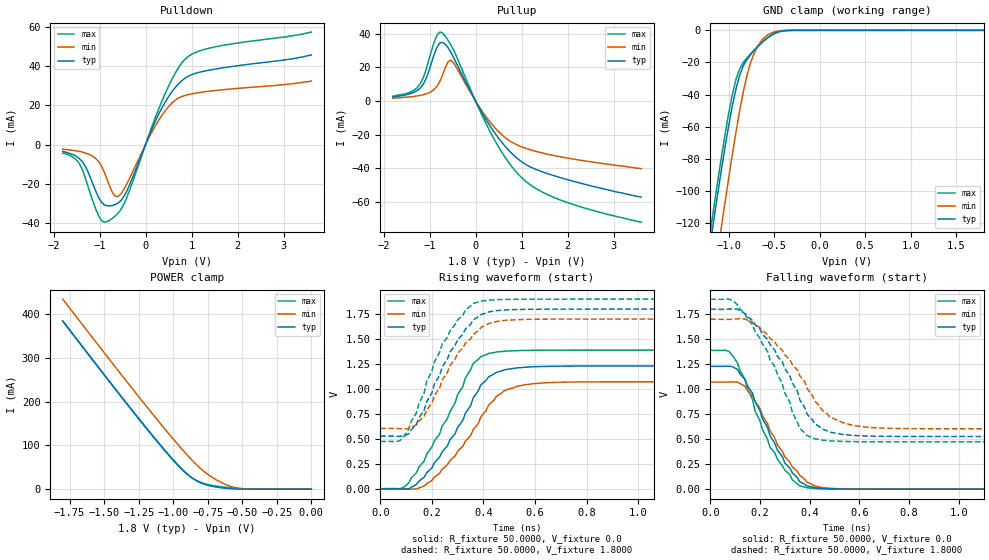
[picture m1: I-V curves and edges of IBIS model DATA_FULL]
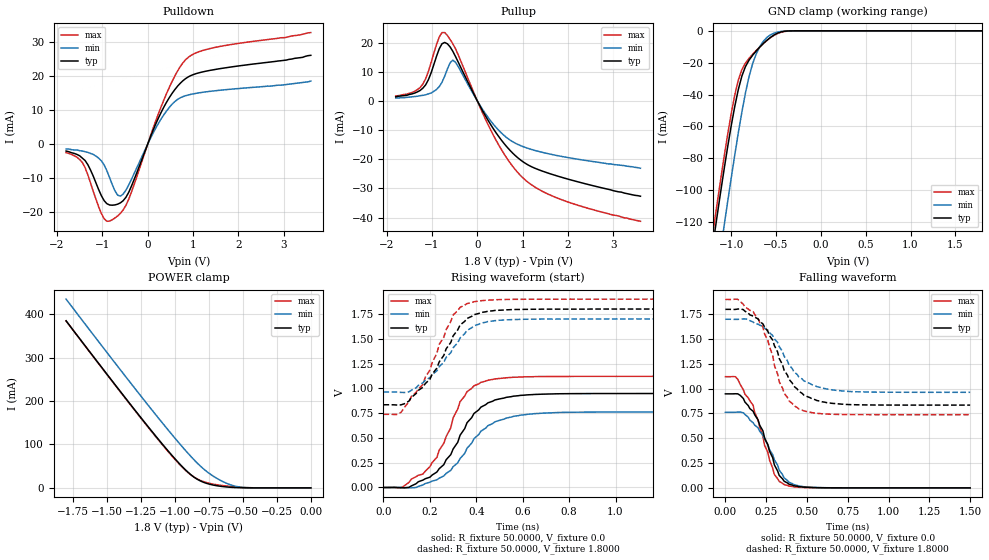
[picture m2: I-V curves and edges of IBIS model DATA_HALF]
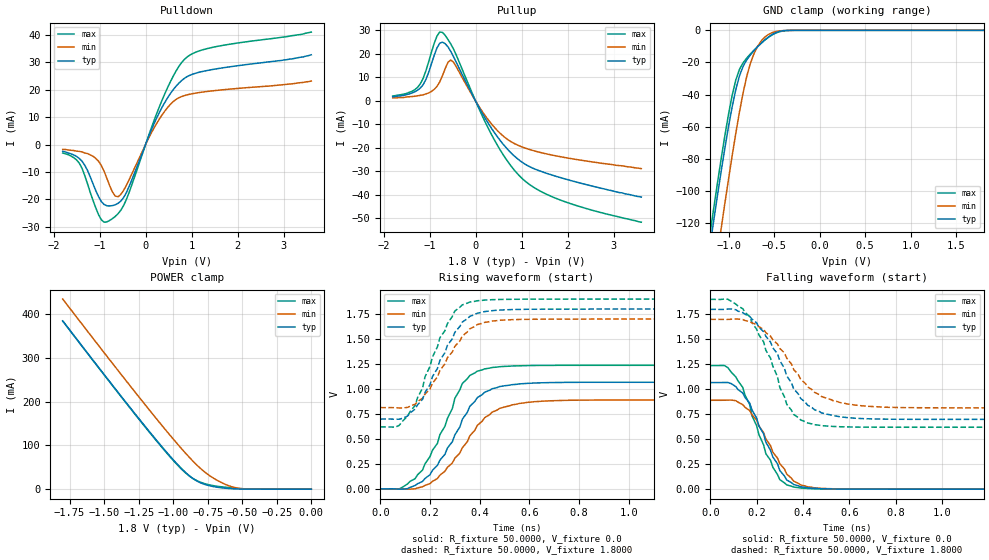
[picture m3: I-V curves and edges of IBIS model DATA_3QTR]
| IBIS file usesk1g16ac.ibs created by s2ibis3 verion 1.1
| North Carolina State University, ERL, 2006
| This Model is valid for Commercial Temperature Range 0C<=Tc<=70C
| Valid for LPDDR-333/400 operation
| Part Number   VDD/VDDQ   Package   Architecture
| SCE18K1G160AF   1.8 +0.1/-0.1  60-Ball FBGA   64Meg x 16
[IBIS Ver]   3.2
[File name]  usesk1g16ac.ibs
[File Rev]   1.2
[Date]   2015-10-27
[Source]   Simulation of a silicon level SPICE model
[Notes]   IBIS Characteristics for I/O Buffer
   IBIS Model Revision History:
Rev 1.1: 2015-10-27
   - IBIS model file initial creation
Rev 1.2: 2016-10-27
   - Updata company and other informations
[disclaimer] The IBIS models are for modeling purpose only and are
   subject to change without any notice. UniIC is not
   responsible for any problems the models may cause.
[Copyright]  Copyright 2015 UniIC Semiconductors Corp. All rights reserved
|   Component SCE18K1G160AF
[Component]   SCE18K1G160AF
[Manufacturer]  UniIC Semiconductors Corp.
| All balls excluding NC, POWER and GND (R[Ohm], L[H], C[F])
[Package]   | 60-Ball FBGA
|Variable   typ   min   max
R_pkg   366m   250m   672m
L_pkg   1.68n   1.12n   2.83n
C_pkg   0.31p   0.20p   0.55p
[Pin]   signal_name model_name   R_pin   L_pin   C_pin
A1   VSS   GND
A2   DQ15   DQ   374m   1.51n   0.32p
A3   VSSQ   GND
A7   VDDQ   POWER
A8   DQ0   DQ   390m   1.48n   0.35p
A9   VDD   POWER
B2   DQ13   DQ   444m   2n   0.4p
B3   DQ14   DQ   332m   1.35n   0.29p
B7   DQ1   DQ   268m   1.19n   0.25p
B8   DQ2   DQ   410m   1.6n   0.37p
B9   VSSQ   GND
C1   VSSQ   GND
C2   DQ11   DQ   370m   1.5n   0.34p
C3   DQ12   DQ   318m   1.58n   0.29p
C7   DQ3   DQ   294m   1.27n   0.28p
C8   DQ4   DQ   387m   1.66n   0.36p
C9   VDDQ   POWER
D1   VDDQ   POWER
D2   DQ9   DQ   391m   1.83n   0.33p
D3   DQ10   DQ   267m   1.14n   0.24p
D7   DQ5   DQ   250m   1.12n   0.27p
D8   DQ6   DQ   405m   1.87n   0.32p
D9   VSSQ   GND
E1   VSSQ   GND
E2   UDQS   DQ   406m   1.72n   0.37p
E3   DQ8   DQ   276m   1.28n   0.25p
E7   DQ7   DQ   275m   1.47n   0.21p
E8   LDQS   DQ   395m   1.59n   0.32p
E9   VDDQ   POWER
F1   VSS   GND
F2   UDM   DATA_RCV   388m   1.82n   0.32p
F7   A13   CLKCA_RCV   264m   1.18n   0.24p
F8   LDM   DATA_RCV   398m   1.54n   0.36p
F9   VDD   POWER
G1   CKE   CLKCA_RCV   453m   2.62n   0.36p
G2   CK   CLKCA_RCV   364m   1.97n   0.32p
G3   CK#   CLKCA_RCV   353m   1.72n   0.25p
G7   WE#   CLKCA_RCV   284m   1.32n   0.26p
G8   CAS#   CLKCA_RCV   381m   1.69n   0.35p
G9   RAS#   CLKCA_RCV   474m   2.32n   0.4p
H1   A9   CLKCA_RCV   457m   2.73n   0.33p
H2   A11   CLKCA_RCV   388m   2.17n   0.29p
H3   A12   CLKCA_RCV   263m   1.36n   0.25p
H7   CS#   CLKCA_RCV   262m   1.22n   0.24p
H8   BA0   CLKCA_RCV   394m   1.67n   0.36p
H9   BA1   CLKCA_RCV   508m   2.19n   0.42p
J1   A6   CLKCA_RCV   672m   2.79n   0.55p
J2   A7   CLKCA_RCV   380m   1.64n   0.3p
J3   A8   CLKCA_RCV   253m   1.34n   0.2p
J7   A10   CLKCA_RCV   263m   1.28n   0.22p
J8   A0   CLKCA_RCV   364m   1.68n   0.29p
J9   A1   CLKCA_RCV   661m   2.83n   0.54p
K1   VSS   GND
K2   A4   CLKCA_RCV   412m   1.87n   0.34p
K3   A5   CLKCA_RCV   266m   1.3n   0.23p
K7   A2   CLKCA_RCV   250m   1.18n   0.24p
K8   A3   CLKCA_RCV   367m   1.75n   0.31p
K9   VDD   POWER
|*****************************  Diff Pin  *************************************
[Diff Pin]  inv_pin  vdiff   tdelay_typ  tdelay_min  tdelay_max
G2   G3   1.08V   NA   NA   NA
|*****************************  Model Selector ********************************
[Model Selector]   DQ
DATA_FULL   Full-Strength Output Driver
DATA_3QTR   75% Strength Output Driver
DATA_HALF   Half-Strength Output Driver
DATA_RCV   Data/Data Strobe/Data Mask Receiver
| Models and submodels in the file (5): DATA_FULL (I/O), DATA_HALF (I/O), DATA_3QTR (I/O), DATA_RCV (Input), CLKCA_RCV (Input)
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|   Model DATA_FULL
[Model]  DATA_FULL
Model_type   I/O
Polarity   Non-Inverting
Enable   Active-High
Vinl  = 360.000mV
Vinh  = 1440.000mV
Vmeas = 900.000mV
Cref  = 20.000pF
C_comp   2.0990pF   2.0750pF   2.3110pF
[Temperature Range]   25.0000   70.0000   0.0
[Voltage Range]   1.8000V   1.7000V   1.9000V
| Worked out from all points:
|   slope of the pulldown table from 0 to 0.27 V, typ, clamps not added: 18.2 ohm
|   slope of the pullup table from 0 to 0.27 V, typ, clamps not added: 21 ohm
|   GND clamp passes 1 mA (typ) near -0.46 V on its own axis
|   POWER clamp passes 1 mA (typ) near -0.57 V on its own axis
|   rising waveform, R_fixture 50.0000, V_fixture 0.0: 20-80 % time 173ps typ, 179ps min, 160ps max; typ from 0 V to 1.23 V
|   rising waveform, R_fixture 50.0000, V_fixture 1.8000: 20-80 % time 150ps typ, 150ps min, 141ps max; typ from 0.527 V to 1.8 V
|   falling waveform, R_fixture 50.0000, V_fixture 0.0: 20-80 % time 143ps typ, 148ps min, 140ps max; typ from 1.23 V to 0 V
|   falling waveform, R_fixture 50.0000, V_fixture 1.8000: 20-80 % time 174ps typ, 187ps min, 158ps max; typ from 1.8 V to 0.527 V
[Pulldown]
|Voltage   I(typ)   I(min)   I(max)
-1.8V     -3.5mA     -2.4mA     -4.4mA
-1.44V    -7.2mA     -3.5mA     -9.6mA
-1.26V    -13.5mA    -4.7mA     -20.7mA
-1.02V    -27.06mA   -8.7mA     -36.42mA
-840mV    -31.35mA   -17.64mA   -39.44mA
-660mV    -30.74mA   -26.42mA   -36.6mA
-540mV    -28.79mA   -25.39mA   -33.36mA
360mV     18.94mA    15.09mA    22.48mA
660mV     29.6mA     22.96mA    37.15mA
900mV     34.59mA    25.38mA    44.54mA
1.56V     38.77mA    27.72mA    50.17mA
3.6V      45.8mA     32.5mA     57.5mA
[Pullup]
|Voltage   I(typ)   I(min)   I(max)
-1.8V     2.5mA      1.7mA      2.9mA
-1.26V    6.4mA      3.1mA      8.2mA
-1.08V    13.03mA    4.3mA      18.27mA
-840mV    31.99mA    8.72mA     39.09mA
-720mV    34.94mA    15.29mA    40.57mA
-600mV    31.88mA    23.25mA    36.23mA
-540mV    29.17mA    24.33mA    33.62mA
360mV     -16.7mA    -14.04mA   -20.48mA
720mV     -29.32mA   -23.3mA    -36.55mA
1.02V     -36.51mA   -27.44mA   -46.11mA
1.92V     -46.19mA   -33.57mA   -59.68mA
3.6V      -57.2mA    -40.3mA    -72.1mA
[GND_clamp]
|Voltage   I(typ)   I(min)   I(max)
-1.8V     -382.1mA   -420.9mA   -375.5mA
-1.2V     -133.2mA   -170.8mA   -125.6mA
-1.16V    -117.7mA   -154.8mA   -110mA
-1.08V    -87.61mA   -123.2mA   -79.77mA
-1V       -59.95mA   -92.78mA   -52.3mA
-920mV    -36.92mA   -64.12mA   -30.96mA
-880mV    -28.39mA   -50.93mA   -24.34mA
-800mV    -18.4mA    -28.71mA   -17.29mA
-680mV    -10.16mA   -9.871mA   -10.08mA
-560mV    -4.068mA   -2.483mA   -4.273mA
-320mV    -22.85uA   -25.25uA   -54.98uA
1.8V      3.312nA    24.23nA    3.394nA
[POWER_clamp]
|Voltage   I(typ)   I(min)   I(max)
-1.8V     384.7mA    434.6mA    384.4mA
-1.4V     221.6mA    271.6mA    220.8mA
-1.14V    119.1mA    168.3mA    117.7mA
-960mV    53.65mA    99.93mA    52.25mA
-900mV    35.09mA    78.55mA    34.34mA
-860mV    24.89mA    65.06mA    25.09mA
-800mV    14.21mA    46.71mA    15.61mA
-720mV    6.601mA    27.45mA    8.67mA
-640mV    2.692mA    13.43mA    5.023mA
-560mV    790.7uA    4.166mA    2.388mA
-440mV    59.56uA    254.6uA    284uA
0V        3.312nA    8.237nA    3.878nA
[Ramp]
| variable   typ   min   max
dV/dt_r  0.7374/0.1699n   0.6426/0.1795n   0.8334/0.1648n
dV/dt_f  0.7638/0.1717n   0.6576/0.1866n   0.8558/0.1598n
R_load = 50.0000
[Rising Waveform]
R_fixture= 50.0000
V_fixture= 0.0
V_fixture_min= 0.0
V_fixture_max= 0.0
|time   V(typ)   V(min)   V(max)
0s        0V         0V         0V
90.91ps   -4.216mV   -497.2uV   15.11mV
140ps     41.75mV    -2.255mV   158.6mV
170ps     115mV      26.85mV    275.9mV
290ps     551.3mV    327.8mV    860.2mV
360ps     908.9mV    590.6mV    1.254V
420ps     1.121V     838.2mV    1.355V
480ps     1.191V     980.7mV    1.378V
590ps     1.222V     1.052V     1.387V
1.5ns     1.229V     1.071V     1.389V
[Rising Waveform]
R_fixture= 50.0000
V_fixture= 1.8000
V_fixture_min= 1.7000
V_fixture_max= 1.9000
|time   V(typ)   V(min)   V(max)
0s        527mV      604mV      473.6mV
75.76ps   524.6mV    601.8mV    480.6mV
140ps     646.7mV    638.8mV    759.9mV
200ps     959.8mV    857mV      1.179V
240ps     1.22V      1.089V     1.452V
300ps     1.494V     1.357V     1.692V
360ps     1.69V      1.544V     1.855V
420ps     1.771V     1.655V     1.889V
520ps     1.794V     1.692V     1.897V
1.5ns     1.8V       1.7V       1.9V
[Falling Waveform]
R_fixture= 50.0000
V_fixture= 0.0
V_fixture_min= 0.0
V_fixture_max= 0.0
|time   V(typ)   V(min)   V(max)
0s        1.229V     1.071V     1.389V
75.76ps   1.231V     1.072V     1.377V
110ps     1.197V     1.07V      1.259V
170ps     959.1mV    934.7mV    898.6mV
180ps     877.9mV    875.6mV    781.7mV
240ps     535.2mV    582.8mV    419.7mV
300ps     261.6mV    322.9mV    189.5mV
360ps     74.58mV    138.3mV    32.52mV
480ps     4.177mV    8.446mV    1.931mV
1.5ns     0V         -795nV     0V
[Falling Waveform]
R_fixture= 50.0000
V_fixture= 1.8000
V_fixture_min= 1.7000
V_fixture_max= 1.9000
|time   V(typ)   V(min)   V(max)
0s        1.8V       1.7V       1.9V
90.91ps   1.805V     1.7V       1.884V
170ps     1.688V     1.669V     1.646V
290ps     1.273V     1.388V     1.053V
350ps     982.2mV    1.193V     673.8mV
360ps     894.7mV    1.136V     607mV
420ps     655.1mV    883.1mV    504.4mV
480ps     571.5mV    724.7mV    483.2mV
620ps     532.4mV    622mV      474.5mV
1.5ns     527mV      604mV      473.6mV
|   Model DATA_HALF
[Model]  DATA_HALF
Model_type   I/O
Polarity   Non-Inverting
Enable   Active-High
Vinl  = 360.000mV
Vinh  = 1440.000mV
Vmeas = 900.000mV
Cref  = 20.000pF
C_comp   2.0990pF   2.0750pF   2.3110pF
[Temperature Range]   25.0000   70.0000   0.0
[Voltage Range]   1.8000V   1.7000V   1.9000V
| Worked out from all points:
|   slope of the pulldown table from 0 to 0.27 V, typ, clamps not added: 31.3 ohm
|   slope of the pullup table from 0 to 0.27 V, typ, clamps not added: 36.1 ohm
|   GND clamp passes 1 mA (typ) near -0.46 V on its own axis
|   POWER clamp passes 1 mA (typ) near -0.57 V on its own axis
|   rising waveform, R_fixture 50.0000, V_fixture 0.0: 20-80 % time 156ps typ, 168ps min, 137ps max; typ from 0 V to 0.948 V
|   rising waveform, R_fixture 50.0000, V_fixture 1.8000: 20-80 % time 149ps typ, 150ps min, 145ps max; typ from 0.834 V to 1.8 V
|   falling waveform, R_fixture 50.0000, V_fixture 0.0: 20-80 % time 140ps typ, 145ps min, 140ps max; typ from 0.948 V to 0 V
|   falling waveform, R_fixture 50.0000, V_fixture 1.8000: 20-80 % time 172ps typ, 179ps min, 146ps max; typ from 1.8 V to 0.834 V
[Pulldown]
|Voltage   I(typ)   I(min)   I(max)
-1.8V     -2mA       -1.4mA     -2.5mA
-1.44V    -4.1mA     -2mA       -5.4mA
-1.02V    -15.18mA   -4.9mA     -20.41mA
-840mV    -17.9mA    -9.82mA    -22.65mA
-660mV    -17.64mA   -15.01mA   -21.1mA
-540mV    -16.62mA   -14.68mA   -19.34mA
-360mV    -12.42mA   -10.4mA    -14.2mA
300mV     9.454mA    7.512mA    11.15mA
600mV     16.1mA     12.58mA    20.1mA
840mV     19.36mA    14.31mA    24.93mA
1.44V     21.91mA    15.68mA    28.39mA
3.6V      26.2mA     18.6mA     32.9mA
[Pullup]
|Voltage   I(typ)   I(min)   I(max)
-1.8V     1.4mA      1mA        1.7mA
-1.38V    2.7mA      1.5mA      3.3mA
-1.2V     4.4mA      1.9mA      5.8mA
-1.08V    7.23mA     2.4mA      10.07mA
-840mV    17.87mA    4.9mA      21.91mA
-720mV    20.06mA    8.48mA     23.44mA
-600mV    18.52mA    13.08mA    21.06mA
-480mV    15.19mA    13.26mA    17.84mA
360mV     -9.695mA   -8.123mA   -11.94mA
1.02V     -21.01mA   -15.74mA   -26.6mA
1.86V     -26.2mA    -19.05mA   -33.89mA
3.6V      -32.7mA    -23.1mA    -41.3mA
[GND_clamp]
|Voltage   I(typ)   I(min)   I(max)
-1.8V     -382.1mA   -420.9mA   -375.5mA
-1.2V     -133.2mA   -170.8mA   -125.6mA
-1.16V    -117.7mA   -154.8mA   -110mA
-1.08V    -87.61mA   -123.2mA   -79.77mA
-1V       -59.95mA   -92.78mA   -52.3mA
-920mV    -36.92mA   -64.12mA   -30.96mA
-880mV    -28.39mA   -50.93mA   -24.34mA
-800mV    -18.4mA    -28.71mA   -17.29mA
-680mV    -10.16mA   -9.871mA   -10.08mA
-560mV    -4.068mA   -2.483mA   -4.273mA
-320mV    -22.85uA   -25.25uA   -54.98uA
1.8V      3.312nA    24.23nA    3.394nA
[POWER_clamp]
|Voltage   I(typ)   I(min)   I(max)
-1.8V     384.7mA    434.6mA    384.4mA
-1.4V     221.6mA    271.6mA    220.8mA
-1.14V    119.1mA    168.3mA    117.7mA
-960mV    53.65mA    99.93mA    52.25mA
-900mV    35.09mA    78.55mA    34.34mA
-860mV    24.89mA    65.06mA    25.09mA
-800mV    14.21mA    46.71mA    15.61mA
-720mV    6.601mA    27.45mA    8.67mA
-640mV    2.692mA    13.43mA    5.023mA
-560mV    790.7uA    4.166mA    2.388mA
-440mV    59.56uA    254.6uA    284uA
0V        3.312nA    8.237nA    3.878nA
[Ramp]
| variable   typ   min   max
dV/dt_r  0.5687/0.1549n   0.4570/0.1668n   0.6726/0.1381n
dV/dt_f  0.5793/0.1729n   0.4419/0.1794n   0.6973/0.1449n
R_load = 50.0000
[Rising Waveform]
R_fixture= 50.0000
V_fixture= 0.0
V_fixture_min= 0.0
V_fixture_max= 0.0
|time   V(typ)   V(min)   V(max)
0s        0V         0V         0V
75.76ps   -2.229mV   491.3uV    -1.644mV
200ps     103.9mV    53.19mV    210mV
260ps     230.8mV    117mV      446.2mV
330ps     527.3mV    292.8mV    866mV
360ps     653.7mV    396.5mV    967mV
420ps     811mV      568.5mV    1.061V
530ps     909.9mV    701mV      1.107V
650ps     938.4mV    744.7mV    1.118V
1.5ns     947.9mV    761.7mV    1.121V
[Rising Waveform]
R_fixture= 50.0000
V_fixture= 1.8000
V_fixture_min= 1.7000
V_fixture_max= 1.9000
|time   V(typ)   V(min)   V(max)
0s        834.5mV    963.5mV    737.9mV
75.76ps   833.5mV    959.1mV    758.7mV
170ps     1.011V     1.056V     1.039V
230ps     1.204V     1.176V     1.353V
240ps     1.267V     1.218V     1.444V
300ps     1.529V     1.41V      1.74V
360ps     1.705V     1.585V     1.855V
420ps     1.765V     1.658V     1.884V
530ps     1.792V     1.691V     1.897V
1.5ns     1.8V       1.7V       1.9V
[Falling Waveform]
R_fixture= 50.0000
V_fixture= 0.0
V_fixture_min= 0.0
V_fixture_max= 0.0
|time   V(typ)   V(min)   V(max)
0s        947.9mV    761.7mV    1.121V
60.61ps   948.9mV    762.2mV    1.121V
110ps     900.9mV    757mV      989.3mV
170ps     772.5mV    656.6mV    832.2mV
230ps     574.9mV    532.6mV    519.2mV
240ps     505.7mV    488.2mV    428.9mV
300ps     232mV      282.8mV    135.1mV
360ps     67.03mV    100.4mV    33.3mV
530ps     3.545mV    5.524mV    1.62mV
1.5ns     0V         0V         0V
[Falling Waveform]
R_fixture= 50.0000
V_fixture= 1.8000
V_fixture_min= 1.7000
V_fixture_max= 1.9000
|time   V(typ)   V(min)   V(max)
0s        1.8V       1.7V       1.9V
75.76ps   1.803V     1.699V     1.901V
200ps     1.704V     1.65V      1.706V
290ps     1.49V      1.535V     1.334V
330ps     1.304V     1.424V     1.07V
360ps     1.186V     1.326V     954.2mV
450ps     973.6mV    1.119V     796.2mV
560ps     880.9mV    1.021V     751.4mV
710ps     844.3mV    978mV      739.7mV
1.5ns     834.5mV    963.5mV    737.9mV
|   Model DATA_3QTR
[Model]  DATA_3QTR
Model_type   I/O
Polarity   Non-Inverting
Enable   Active-High
Vinl  = 360.000mV
Vinh  = 1440.000mV
Vmeas = 900.000mV
Cref  = 20.000pF
C_comp   2.0990pF   2.0750pF   2.3110pF
[Temperature Range]   25.0000   70.0000   0.0
[Voltage Range]   1.8000V   1.7000V   1.9000V
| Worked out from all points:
|   slope of the pulldown table from 0 to 0.27 V, typ, clamps not added: 25.2 ohm
|   slope of the pullup table from 0 to 0.27 V, typ, clamps not added: 29 ohm
|   GND clamp passes 1 mA (typ) near -0.46 V on its own axis
|   POWER clamp passes 1 mA (typ) near -0.57 V on its own axis
|   rising waveform, R_fixture 50.0000, V_fixture 0.0: 20-80 % time 151ps typ, 159ps min, 140ps max; typ from 0 V to 1.07 V
|   rising waveform, R_fixture 50.0000, V_fixture 1.8000: 20-80 % time 131ps typ, 132ps min, 123ps max; typ from 0.699 V to 1.8 V
|   falling waveform, R_fixture 50.0000, V_fixture 0.0: 20-80 % time 125ps typ, 132ps min, 122ps max; typ from 1.07 V to 0 V
|   falling waveform, R_fixture 50.0000, V_fixture 1.8000: 20-80 % time 159ps typ, 179ps min, 139ps max; typ from 1.8 V to 0.699 V
[Pulldown]
|Voltage   I(typ)   I(min)   I(max)
-1.8V     -2.5mA     -1.8mA     -3.1mA
-1.44V    -5.1mA     -2.5mA     -6.8mA
-1.02V    -19.09mA   -6.1mA     -25.69mA
-840mV    -22.38mA   -12.38mA   -28.27mA
-660mV    -22.02mA   -18.8mA    -26.3mA
-540mV    -20.71mA   -18.28mA   -24.06mA
-360mV    -15.41mA   -12.92mA   -17.61mA
300mV     11.75mA    9.345mA    13.83mA
600mV     20.05mA    15.68mA    24.98mA
840mV     24.15mA    17.87mA    31.06mA
1.5V      27.55mA    19.71mA    35.68mA
3.6V      32.8mA     23.2mA     41.1mA
[Pullup]
|Voltage   I(typ)   I(min)   I(max)
-1.8V     1.8mA      1.3mA      2.1mA
-1.38V    3.4mA      1.9mA      4.1mA
-1.2V     5.5mA      2.4mA      7.3mA
-1.08V    9.13mA     3mA        12.77mA
-840mV    22.51mA    6.16mA     27.58mA
-720mV    25.04mA    10.7mA     29.2mA
-600mV    23.03mA    16.44mA    26.17mA
-480mV    18.86mA    16.49mA    22.13mA
360mV     -12.05mA   -10.11mA   -14.82mA
1.02V     -26.2mA    -19.65mA   -33.15mA
1.92V     -33.06mA   -24.01mA   -42.74mA
3.6V      -40.9mA    -28.8mA    -51.6mA
[GND_clamp]
|Voltage   I(typ)   I(min)   I(max)
-1.8V     -382.1mA   -420.9mA   -375.5mA
-1.2V     -133.2mA   -170.8mA   -125.6mA
-1.16V    -117.7mA   -154.8mA   -110mA
-1.08V    -87.61mA   -123.2mA   -79.77mA
-1V       -59.95mA   -92.78mA   -52.3mA
-920mV    -36.92mA   -64.12mA   -30.96mA
-880mV    -28.39mA   -50.93mA   -24.34mA
-800mV    -18.4mA    -28.71mA   -17.29mA
-680mV    -10.16mA   -9.871mA   -10.08mA
-560mV    -4.068mA   -2.483mA   -4.273mA
-320mV    -22.85uA   -25.25uA   -54.98uA
1.8V      3.312nA    24.23nA    3.394nA
[POWER_clamp]
|Voltage   I(typ)   I(min)   I(max)
-1.8V     384.7mA    434.6mA    384.4mA
-1.4V     221.6mA    271.6mA    220.8mA
-1.14V    119.1mA    168.3mA    117.7mA
-960mV    53.65mA    99.93mA    52.25mA
-900mV    35.09mA    78.55mA    34.34mA
-860mV    24.89mA    65.06mA    25.09mA
-800mV    14.21mA    46.71mA    15.61mA
-720mV    6.601mA    27.45mA    8.67mA
-640mV    2.692mA    13.43mA    5.023mA
-560mV    790.7uA    4.166mA    2.388mA
-440mV    59.56uA    254.6uA    284uA
0V        3.312nA    8.237nA    3.878nA
[Ramp]
| variable   typ   min   max
dV/dt_r  0.6402/0.1506n   0.5339/0.1638n   0.7422/0.1356n
dV/dt_f  0.6607/0.1623n   0.5318/0.1784n   0.7681/0.1395n
R_load = 50.0000
[Rising Waveform]
R_fixture= 50.0000
V_fixture= 0.0
V_fixture_min= 0.0
V_fixture_max= 0.0
|time   V(typ)   V(min)   V(max)
0s        0V         0V         0V
90.91ps   -3.003mV   -1.061mV   18.97mV
140ps     33.44mV    628.7uV    101.8mV
200ps     141.5mV    52.45mV    323.3mV
290ps     472.6mV    259.4mV    804.8mV
330ps     696.5mV    411.5mV    1.055V
390ps     913mV      634.7mV    1.178V
480ps     1.024V     805.5mV    1.223V
620ps     1.06V      872.7mV    1.235V
1.5ns     1.067V     889.9mV    1.237V
[Rising Waveform]
R_fixture= 50.0000
V_fixture= 1.8000
V_fixture_min= 1.7000
V_fixture_max= 1.9000
|time   V(typ)   V(min)   V(max)
0s        698.8mV    813.6mV    619.8mV
75.76ps   697.5mV    809.8mV    635mV
140ps     797.7mV    847.7mV    834.3mV
200ps     1.042V     1V         1.226V
240ps     1.287V     1.186V     1.514V
300ps     1.568V     1.427V     1.781V
360ps     1.727V     1.602V     1.87V
420ps     1.775V     1.667V     1.89V
530ps     1.795V     1.694V     1.898V
1.5ns     1.8V       1.7V       1.9V
[Falling Waveform]
R_fixture= 50.0000
V_fixture= 0.0
V_fixture_min= 0.0
V_fixture_max= 0.0
|time   V(typ)   V(min)   V(max)
0s        1.067V     889.9mV    1.237V
75.76ps   1.068V     891.6mV    1.217V
140ps     963.2mV    847.2mV    1.019V
200ps     711.8mV    692.2mV    634.9mV
240ps     470mV      500.9mV    354.3mV
300ps     186.4mV    255.6mV    95.45mV
330ps     92.05mV    151mV      42.65mV
390ps     24.43mV    42.73mV    11.12mV
480ps     4.545mV    7.823mV    2.072mV
1.5ns     0V         0V         0V
[Falling Waveform]
R_fixture= 50.0000
V_fixture= 1.8000
V_fixture_min= 1.7000
V_fixture_max= 1.9000
|time   V(typ)   V(min)   V(max)
0s        1.8V       1.7V       1.9V
75.76ps   1.803V     1.699V     1.901V
170ps     1.729V     1.677V     1.727V
260ps     1.472V     1.532V     1.311V
330ps     1.134V     1.311V     849.2mV
360ps     1.004V     1.197V     747.9mV
420ps     840.3mV    1.024V     662.4mV
530ps     735.4mV    885.8mV    627.7mV
650ps     707.1mV    835.2mV    621.1mV
1.5ns     698.8mV    813.6mV    619.8mV
